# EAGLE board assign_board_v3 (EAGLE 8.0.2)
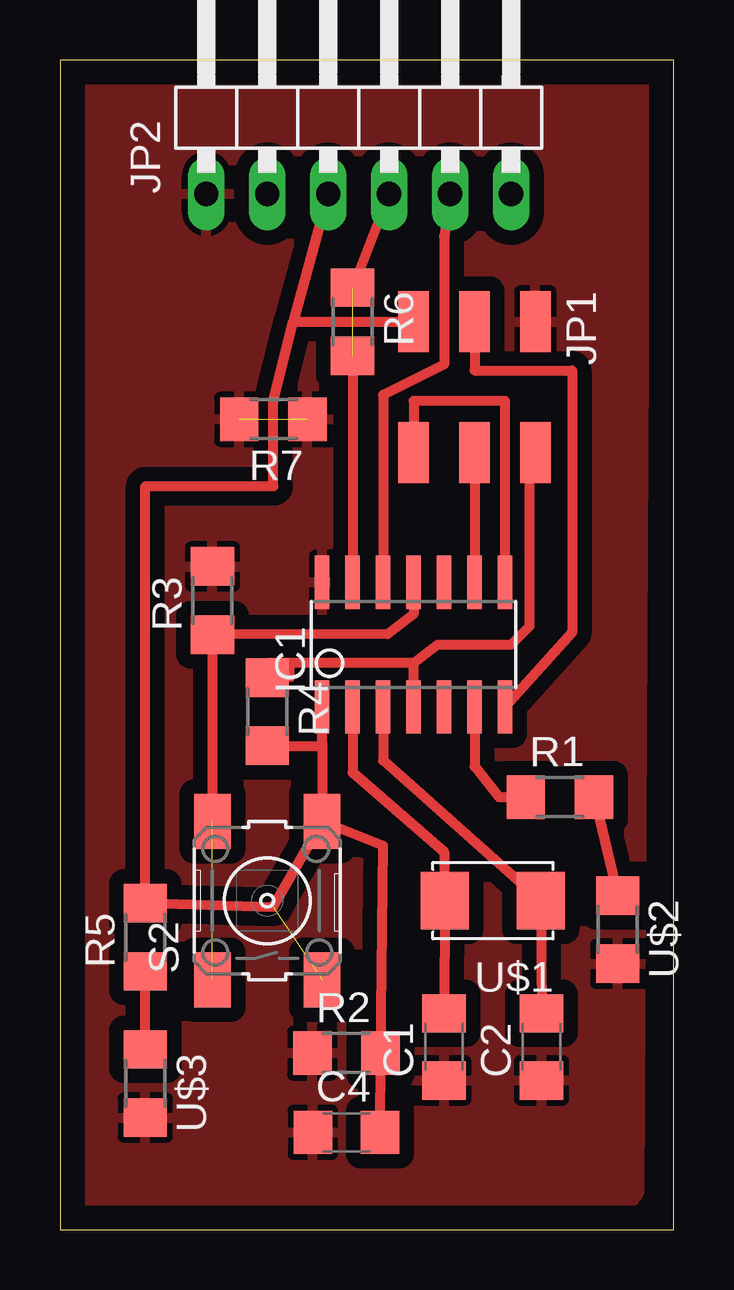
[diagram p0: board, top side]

Size 25.58 x 48.76 mm. Coordinates in mm from the lower left corner, seen from the top.
Outline: 0,0 25.58,0 25.58,48.76 0,48.76 0,0
Copper layers (1*16): Top 0.035mm / dielectric 1.5mm / Bottom 0.035mm
Design rules "assign_board_v3 *": minimum track width 10mil, minimum drill 24mil, track to track 0.205mm, track to pad 0.205mm, pad to pad 0.205mm, via to via 0.205mm, smd to smd 8mil, copper to edge 40mil, drill to drill 8mil, minimum pad ring 10mil, minimum via ring 8mil, stop-mask expansion 4mil, vias tented up to drill 0mil, thermal gap 10mil
Net classes: 0 default: clearance 0.205 mm

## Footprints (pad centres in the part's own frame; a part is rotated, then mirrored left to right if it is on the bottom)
C1206 = smd 1.6 x 1.8: 1 -1.4,0; 2 1.4,0
SOIC14 = smd 0.61 x 2.21: 1 -3.81,-2.603; 2 -2.54,-2.603; 3 -1.27,-2.603; 4 0,-2.603; 5 1.27,-2.603; 6 2.54,-2.603; 7 3.81,-2.603; 8 3.81,2.603; 9 2.54,2.603; 10 1.27,2.603; 11 0,2.603; 12 -1.27,2.603; 13 -2.54,2.603; 14 -3.81,2.603
2X03SMD = smd 2.54 x 1.27: 1 -2.54,2.54; 2 2.92,2.54; 3 -2.54,0; 4 2.92,0; 5 -2.54,-2.54; 6 2.92,-2.54
1X06/90 = drill 1.016 long: 1 -6.35,-3.81; 2 -3.81,-3.81; 3 -1.27,-3.81; 4 1.27,-3.81; 5 3.81,-3.81; 6 6.35,-3.81
R1206 = smd 1.6 x 1.803: 1 -1.422,0; 2 1.422,0
6MM_SWITCH = smd 2.286 x 1.524: 1 -3.302,2.286; 2 3.302,2.286; 3 -3.302,-2.286; 4 3.302,-2.286
2-SMD-5X3MM = smd 2 x 2.4: P$1 -2,0; P$2 2,0
LED1206 = smd 1.6 x 1.803: 1 -1.422,0; 2 1.422,0

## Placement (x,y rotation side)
C1  22p  [C1206]  16,7.62 90 top
C2  22p  [C1206]  20.07,7.62 90 top
C4  1u  [C1206]  11.94,4.06 0 top
IC1  ATTINY44-SSU  [SOIC14]  14.73,24.38 0 top
JP1  P6  [2X03SMD]  17.27,35.31 270 top
JP2  6  [1X06/90]  12.45,46.99 0 top
R1  499  [R1206]  20.83,18.03 0 top
R2  10k  [R1206]  11.94,7.37 0 top
R3  0  [R1206]  6.35,26.23 90 top
R4  10k  [R1206]  8.64,21.59 270 top
R5  499  [R1206]  3.56,12.19 90 top
R6  0  [R1206]  12.19,37.85 270 top
R7  0  [R1206]  8.89,33.78 180 top
S2  [6MM_SWITCH]  8.64,13.72 90 top
U$1  CRYSTAL  [2-SMD-5X3MM]  18.03,13.72 180 top
U$2  LED  [LED1206]  23.24,12.51 270 top
U$3  LED  [LED1206]  3.56,6.1 270 top

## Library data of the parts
C1 C2 C4 IC1 JP1 R1-R7 S2 U$1-U$3 = fab
JP2 = pinhead

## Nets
CTS: JP2.2
GND: C1.1 C2.1 C4.1 IC1.14 JP1.1 JP2.1 R2.1 R3.2 R7.1 R7.2 U$2.2 U$3.2
INT0: IC1.13 JP2.4 R6.1 R6.2
MISO: IC1.8 JP1.6
MOSI: IC1.7 JP1.3
N$1: R1.2 U$2.1
N$4: R5.1 U$3.1
PA1: IC1.12 JP2.5
PA2: IC1.11 R3.1 S2.1 S2.2
PA7: IC1.6 R1.1
RST: IC1.4 JP1.2 R4.1
RTS: JP2.6
SCK: IC1.9 JP1.4
VCC: C4.2 IC1.1 JP1.5 JP2.3 R2.2 R4.2 R5.2 S2.3 S2.4
XTAL1: C1.2 IC1.2 U$1.P$2
XTAL2: C2.2 IC1.3 U$1.P$1

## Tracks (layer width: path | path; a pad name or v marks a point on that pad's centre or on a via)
GND  (1 unrouted)
  pour Top (isolate 0.61): 1.78,0.25 0.25,1.52 0.25,47.24 1.52,48.51 23.37,48.51 24.38,47.75 24.13,1.52 23.11,0.25
INT0  (1 unrouted)
  Top 0.406: JP2.4 R6.1 | R6.2 IC1.13
MISO
  Top 0.406: IC1.8 18.54,34.54 14.73,34.54 JP1.6
MOSI
  Top 0.406: JP1.3 17.27,35.81 21.34,35.81 21.34,24.89 IC1.7
N$1
  Top 0.406: R1.2 U$2.1
N$4
  Top 0.406: U$3.1 R5.1
PA1
  Top 0.406: JP2.5 16,41.4 16,36.07 13.46,34.8 IC1.12
PA2  (1 unrouted)
  Top 0.406: S2.2 R3.1 13.65,24.83 14.73,25.65 IC1.11
PA7
  Top 0.406: IC1.6 17.27,19.3 18.29,18.03 R1.1
RST
  Top 0.254: R4.1 9.65,22.96 9.65,23.62
  Top 0.406: IC1.4 14.73,23.62 | 14.73,23.62 15.75,24.38 18.8,24.38 19.56,25.15 19.56,32.64 JP1.2 | 14.73,23.62 8.64,23.62 R4.1
SCK
  Top 0.406: JP1.4 IC1.9
VCC  (1 unrouted)
  Top 0.406: 10.92,20.32 S2.4 | 10.92,20.32 IC1.1 | S2.4 13.46,16 R2.2 C4.2 | JP2.3 9.72,37.85 | 9.72,37.85 JP1.5 | 9.72,37.85 8.89,34.54 8.89,30.99 3.56,30.99 R5.2 8.89,13.46 S2.4 | R4.2 10.92,20.17 10.92,20.32
XTAL1
  Top 0.406: C1.2 U$1.P$2 16,15.75 12.19,19.05 IC1.2
XTAL2
  Top 0.406: C2.2 U$1.P$1 13.46,19.56 IC1.3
